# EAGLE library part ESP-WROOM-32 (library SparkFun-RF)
ESP-WROOM-32D - trace antenna (includes keepout) ESP-WROOM-32U - U.FL antenna connector Includes both "standard" footprints and "narrow" version (for use with tighter layouts).
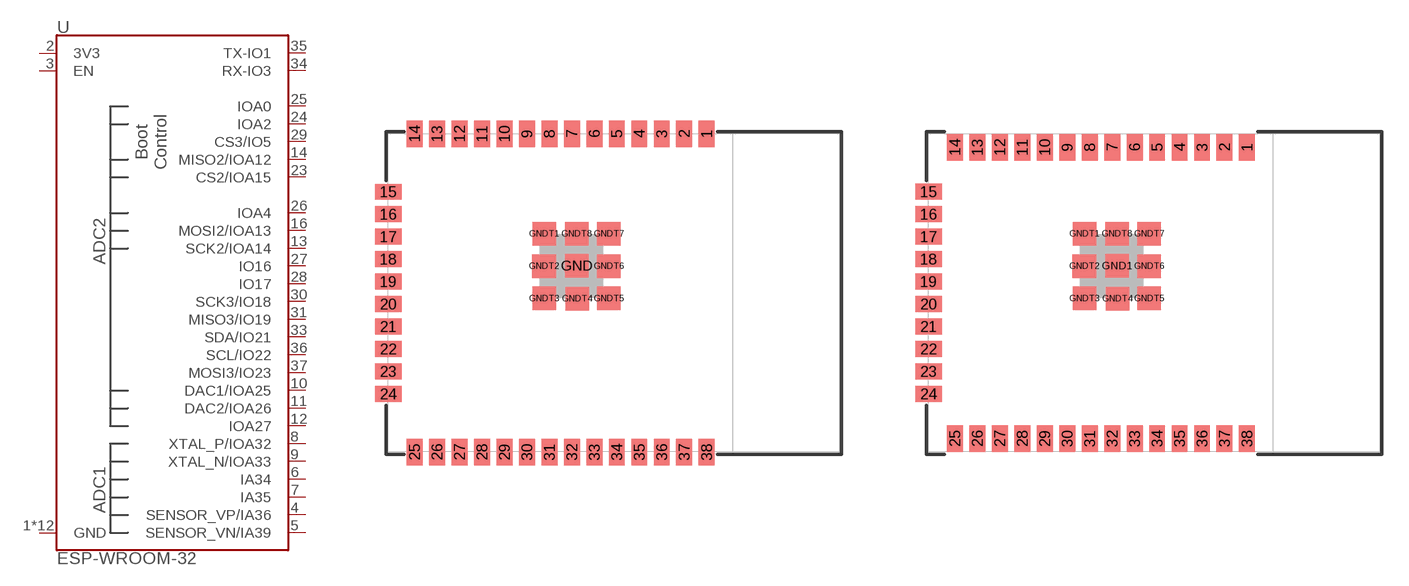
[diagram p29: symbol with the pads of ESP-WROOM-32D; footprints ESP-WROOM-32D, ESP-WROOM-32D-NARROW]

Designator prefix U

## ESP-WROOM-3232D (PROD_ID: IC-15676)  [ESP-WROOM-32D]
1  GND
2  3V3
3  EN
4  SENSOR_VP/IA36
5  SENSOR_VN/IA39
6  IA34
7  IA35
8  XTAL_P/IOA32
9  XTAL_N/IOA33
10  DAC1/IOA25
11  DAC2/IOA26
12  IOA27
13  SCK2/IOA14
14  MISO2/IOA12
15  GND
16  MOSI2/IOA13
23  CS2/IOA15
24  IOA2
25  IOA0
26  IOA4
27  IO16
28  IO17
29  CS3/IO5
30  SCK3/IO18
31  MISO3/IO19
33  SDA/IO21
34  RX-IO3
35  TX-IO1
36  SCL/IO22
37  MOSI3/IO23
38  GND
GND  GND
GNDT1  GND
GNDT2  GND
GNDT3  GND
GNDT4  GND
GNDT5  GND
GNDT6  GND
GNDT7  GND
GNDT8  GND

## ESP-WROOM-3232D-NARROW (PROD_ID: IC-15676)  [ESP-WROOM-32D-NARROW]
1  GND
2  3V3
3  EN
4  SENSOR_VP/IA36
5  SENSOR_VN/IA39
6  IA34
7  IA35
8  XTAL_P/IOA32
9  XTAL_N/IOA33
10  DAC1/IOA25
11  DAC2/IOA26
12  IOA27
13  SCK2/IOA14
14  MISO2/IOA12
15  GND
16  MOSI2/IOA13
23  CS2/IOA15
24  IOA2
25  IOA0
26  IOA4
27  IO16
28  IO17
29  CS3/IO5
30  SCK3/IO18
31  MISO3/IO19
33  SDA/IO21
34  RX-IO3
35  TX-IO1
36  SCL/IO22
37  MOSI3/IO23
38  GND
GND1  GND
GNDT1  GND
GNDT2  GND
GNDT3  GND
GNDT4  GND
GNDT5  GND
GNDT6  GND
GNDT7  GND
GNDT8  GND

## ESP-WROOM-32EU-NARROW (PROD_ID: IC-15442)  [ESP-WROOM-32EU-NARROW]
Pads as for ESP-WROOM-32D

## ESP-WROOM-32EU (PROD_ID: IC-15442)  [ESP-WROOM-32EU]
Pads as for ESP-WROOM-32D

## Footprint ESP-WROOM-32D (pad centres in mm)
ESP-WROOM-32D This version of the module contains an onboard trace-antenna connector. It is virtually identical to the onboard u.FL version (ESP32-WROOM-32U), except it is slightly longer and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
smd 0.9 x 1.5: 1 6.43,9; 2 5.16,9; 3 3.89,9; 4 2.62,9; 5 1.35,9; 6 0.08,9; 7 -1.19,9; 8 -2.46,9; 9 -3.73,9; 10 -5,9; 11 -6.27,9; 12 -7.54,9; 13 -8.81,9; 14 -10.08,9; 25 -10.08,-9; 26 -8.81,-9; 27 -7.54,-9; 28 -6.27,-9; 29 -5,-9; 30 -3.73,-9; 31 -2.46,-9; 32 -1.19,-9; 33 0.08,-9; 34 1.35,-9; 35 2.62,-9; 36 3.89,-9; 37 5.16,-9; 38 6.43,-9
smd 1.5 x 0.9: 15 -11.57,5.715; 16 -11.57,4.445; 17 -11.57,3.175; 18 -11.57,1.905; 19 -11.57,0.635; 20 -11.57,-0.635; 21 -11.57,-1.905; 22 -11.57,-3.175; 23 -11.57,-4.445; 24 -11.57,-5.715
smd 1.33 x 1.33: GND -0.912,1.531; GNDT1 -2.751,3.346; GNDT2 -2.761,1.516; GNDT3 -2.751,-0.314; GNDT4 -0.891,-0.324; GNDT5 0.909,-0.314; GNDT6 0.909,1.516; GNDT7 0.909,3.346; GNDT8 -0.921,3.346

## Footprint ESP-WROOM-32D-NARROW (pad centres in mm)
ESP-WROOM-32D This version of the module contains an onboard trace-antenna connector. It is virtually identical to the onboard u.FL version (ESP32-WROOM-32U), except it is slightly longer and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
smd 0.9 x 1.5: 1 6.43,8.238; 2 5.16,8.238; 3 3.89,8.238; 4 2.62,8.238; 5 1.35,8.238; 6 0.08,8.238; 7 -1.19,8.238; 8 -2.46,8.238; 9 -3.73,8.238; 10 -5,8.238; 11 -6.27,8.238; 12 -7.54,8.238; 13 -8.81,8.238; 14 -10.08,8.238; 25 -10.08,-8.238; 26 -8.81,-8.238; 27 -7.54,-8.238; 28 -6.27,-8.238; 29 -5,-8.238; 30 -3.73,-8.238; 31 -2.46,-8.238; 32 -1.19,-8.238; 33 0.08,-8.238; 34 1.35,-8.238; 35 2.62,-8.238; 36 3.89,-8.238; 37 5.16,-8.238; 38 6.43,-8.238
smd 1.5 x 0.9: 15 -11.57,5.715; 16 -11.57,4.445; 17 -11.57,3.175; 18 -11.57,1.905; 19 -11.57,0.635; 20 -11.57,-0.635; 21 -11.57,-1.905; 22 -11.57,-3.175; 23 -11.57,-4.445; 24 -11.57,-5.715
smd 1.33 x 1.33: GND1 -0.912,1.531; GNDT1 -2.751,3.346; GNDT2 -2.761,1.516; GNDT3 -2.751,-0.314; GNDT4 -0.891,-0.324; GNDT5 0.909,-0.314; GNDT6 0.909,1.516; GNDT7 0.909,3.346; GNDT8 -0.921,3.346

## Footprint ESP-WROOM-32EU-NARROW (pad centres in mm)
ESP-WROOM-32EU This version of the module contains the u.FL antenna connector. It is virtually identical to the onboard trace-antenna version (ESP32-WROOM-32D), except it is slightly shorter and does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
smd 0.9 x 1.5: 1 6.43,8.238; 2 5.16,8.238; 3 3.89,8.238; 4 2.62,8.238; 5 1.35,8.238; 6 0.08,8.238; 7 -1.19,8.238; 8 -2.46,8.238; 9 -3.73,8.238; 10 -5,8.238; 11 -6.27,8.238; 12 -7.54,8.238; 13 -8.81,8.238; 14 -10.08,8.238; 25 -10.08,-8.238; 26 -8.81,-8.238; 27 -7.54,-8.238; 28 -6.27,-8.238; 29 -5,-8.238; 30 -3.73,-8.238; 31 -2.46,-8.238; 32 -1.19,-8.238; 33 0.08,-8.238; 34 1.35,-8.238; 35 2.62,-8.238; 36 3.89,-8.238; 37 5.16,-8.238; 38 6.43,-8.238
smd 1.5 x 0.9: 15 -11.57,5.715; 16 -11.57,4.445; 17 -11.57,3.175; 18 -11.57,1.905; 19 -11.57,0.635; 20 -11.57,-0.635; 21 -11.57,-1.905; 22 -11.57,-3.175; 23 -11.57,-4.445; 24 -11.57,-5.715
smd 1.33 x 1.33: GND -0.912,1.531; GNDT1 -2.751,3.346; GNDT2 -2.761,1.516; GNDT3 -2.751,-0.314; GNDT4 -0.891,-0.324; GNDT5 0.909,-0.314; GNDT6 0.909,1.516; GNDT7 0.909,3.346; GNDT8 -0.921,3.346

## Footprint ESP-WROOM-32EU (pad centres in mm)
ESP-WROOM-32EU This version of the module contains the u.FL antenna connector. It is virtually identical to the onboard trace-antenna version (ESP32-WROOM-32D), except it is slightly shorter and does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
smd 0.9 x 1.5: 1 6.43,9; 2 5.16,9; 3 3.89,9; 4 2.62,9; 5 1.35,9; 6 0.08,9; 7 -1.19,9; 8 -2.46,9; 9 -3.73,9; 10 -5,9; 11 -6.27,9; 12 -7.54,9; 13 -8.81,9; 14 -10.08,9; 25 -10.08,-9; 26 -8.81,-9; 27 -7.54,-9; 28 -6.27,-9; 29 -5,-9; 30 -3.73,-9; 31 -2.46,-9; 32 -1.19,-9; 33 0.08,-9; 34 1.35,-9; 35 2.62,-9; 36 3.89,-9; 37 5.16,-9; 38 6.43,-9
smd 1.5 x 0.9: 15 -11.57,5.715; 16 -11.57,4.445; 17 -11.57,3.175; 18 -11.57,1.905; 19 -11.57,0.635; 20 -11.57,-0.635; 21 -11.57,-1.905; 22 -11.57,-3.175; 23 -11.57,-4.445; 24 -11.57,-5.715
smd 1.33 x 1.33: GND -0.912,1.531; GNDT1 -2.751,3.346; GNDT2 -2.761,1.516; GNDT3 -2.751,-0.314; GNDT4 -0.891,-0.324; GNDT5 0.909,-0.314; GNDT6 0.909,1.516; GNDT7 0.909,3.346; GNDT8 -0.921,3.346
